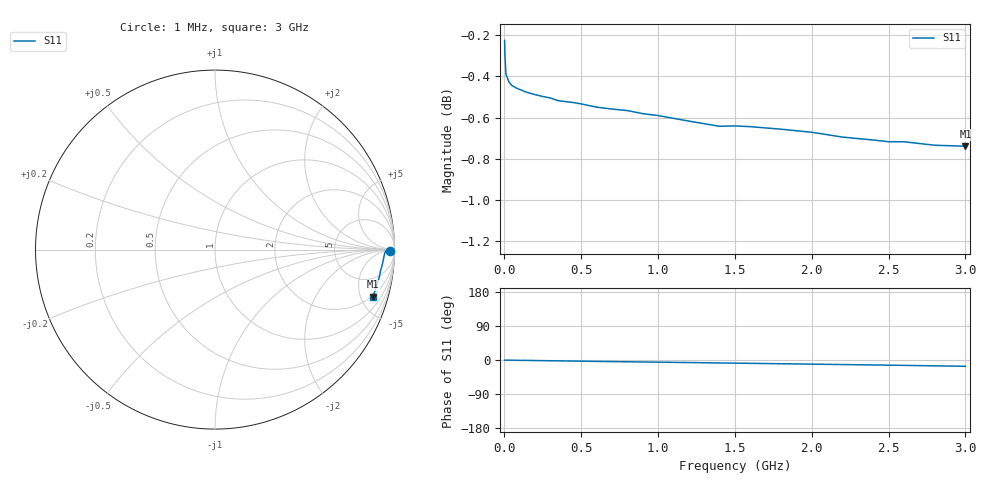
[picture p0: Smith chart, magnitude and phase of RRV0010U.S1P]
! SIEMENS Small Signal Semiconductors
! BA595
! Si PIN Diode in SOD323
! IF = 0.01 mA
! S-Parameters:  July  1992
# GHz  S  MA  R  50
!  f  S11
! GHz  MAG  ANG
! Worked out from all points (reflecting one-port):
!   33 points, 1 MHz to 3 GHz, reference 50 ohm
!   lowest |S11| = -0.7 dB at 3 GHz (marker M1), VSWR 23.51, Z = 94.1 - j315 ohm
!   phase of S11 starts at -0 deg and turns -16 deg over the sweep
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0.001  0.9744 -0.4
0.003  0.9662 -0.5
0.01  0.9561 -0.4
0.03  0.9519 -0.5
0.05  0.95 -0.6
0.06  0.9496 -0.6
0.08  0.9487 -0.8
0.1  0.948 -0.9
0.15  0.9464 -1.1
0.3  0.9435 -2.0
0.35  0.9421 -2.3
0.4  0.9416 -2.5
0.5  0.9404 -3.1
0.6  0.9387 -3.7
0.8  0.9369 -4.7
1  0.9343 -5.7
1.2  0.9314 -6.7
1.4  0.9287 -7.8
1.5  0.9289 -8.3
1.6  0.9285 -8.8
1.8  0.9272 -9.9
2  0.9256 -10.9
2.2  0.9231 -12.0
2.4  0.9216 -13.1
2.5  0.9207 -13.7
2.6  0.9207 -14.2
2.8  0.9189 -15.4
3  0.9184 -16.6
